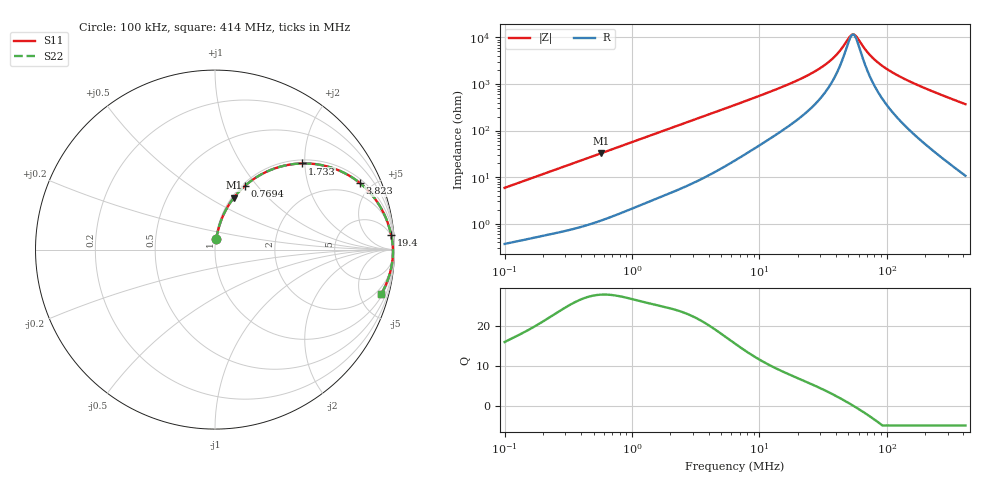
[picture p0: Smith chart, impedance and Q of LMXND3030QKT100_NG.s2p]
! LMXND3030QKT100_NG  S-PARAMETER MODEL  ( General Type )
! Model Generated by TAIYO YUDEN Corporation (https://www.yuden.co.jp/en/)
! Version 1.0
! TAIYO YUDEN Control No. 191023NI43SB-FBB
! Copyright(c) 2019 TAIYO YUDEN CO.,LTD. All Rights Reserved.
! Product Description (link to TY-COMPAS)
! https://ds.yuden.co.jp/TYCOMPAS/or/detail?pn=LMXND3030QKT100MNG&u=M
! Products Name : Inductors
! Characteristics :
!  Inductance : 10 uH , SRF(min) : 28 MHz , DC Resistance(max) : 0.264 Ohm
!  Rated Current : Saturation :700 mA , Temp Rise : 710 mA (40 degC)
!  Case Size : 3.0 x 3.0 / 0.118 x 0.118 [mm/inch] , Thickness : 1.5 / 0.059 [mm/inch]
!  (Conditions: Temperature = 25 degC , DC Bias Current/Voltage = 0A / 0V)
! External Node Assignments :
!  1  o---GGG---o  2
! GND o---------o GND
! Frequency Range : 0.1MHz  -  413.982163MHz  [ 402 STEP ]
# MHz S RI R 50
! Freq[MHz].  S11 Real  S11 Imag  S21 Real  S21 Imag  S12 Real  S12 Imag  S22 Real  S22 Imag
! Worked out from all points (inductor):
!   401 points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, 100 kHz to 414 MHz, reference 50 ohm
!   read as one part in series: L = 9.29 uH near 104.3 kHz
!   highest Q = 27.9 at 574.9 kHz (marker M1), where L = 9.05 uH
!   self-resonance near 53.8 MHz
!   S11 on the Smith chart (normalised r, x): 100 kHz: 1.01, +0.12; 769.4 kHz: 1.03, +0.87; 1.733 MHz: 1.08, +1.93; 3.823 MHz: 1.20, +4.22; 19.4 MHz: 4, +23; 414 MHz: 1.21, -7.38
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0.1  0.00706 0.0581  0.9929 -0.0581  0.9929 -0.0581  0.00706 0.0581
0.211606  0.0201 0.1191  0.9799 -0.1191  0.9799 -0.1191  0.0201 0.1191
0.403501  0.0578 0.2154  0.9422 -0.2154  0.9422 -0.2154  0.0578 0.2154
0.574865  0.105 0.2891  0.895 -0.2891  0.895 -0.2891  0.105 0.2891
0.769415  0.1684 0.3565  0.8316 -0.3565  0.8316 -0.3565  0.1684 0.3565
1.628129  0.4542 0.4784  0.5458 -0.4784  0.5458 -0.4784  0.4542 0.4784
1.73307  0.4835 0.4801  0.5165 -0.4801  0.5165 -0.4801  0.4835 0.4801
2.469096  0.6461 0.4574  0.3539 -0.4574  0.3539 -0.4574  0.6461 0.4574
3.823222  0.8053 0.3724  0.1947 -0.3724  0.1947 -0.3724  0.8053 0.3724
6.434145  0.9128 0.2518  0.0872 -0.2518  0.0872 -0.2518  0.9128 0.2518
19.39728  0.9811 0.0826  0.0189 -0.0826  0.0189 -0.0826  0.9811 0.0826
25.96183  0.9863 0.0555  0.0137 -0.0555  0.0137 -0.0555  0.9863 0.0555
37.76586  0.99 0.0259  0.00999 -0.0259  0.00999 -0.0259  0.99 0.0259
42.79117  0.9907 0.0168  0.00928 -0.0168  0.00928 -0.0168  0.9907 0.0168
50.54681  0.9913 0.00502  0.00868 -0.00502  0.00868 -0.00502  0.9913 0.00502
53.80481  0.9915 0.000618  0.00855 -0.000618  0.00855 -0.000618  0.9915 0.000618
58.47779  0.9916 -0.00527  0.00845 0.00527  0.00845 0.00527  0.9916 -0.00527
69.07654  0.9915 -0.0172  0.00851 0.0172  0.00851 0.0172  0.9915 -0.0172
78.26819  0.9912 -0.0265  0.0088 0.0265  0.0088 0.0265  0.9912 -0.0265
104.7562  0.9896 -0.05  0.0104 0.05  0.0104 0.05  0.9896 -0.05
183.7917  0.9802 -0.1086  0.0198 0.1086  0.0198 0.1086  0.9802 -0.1086
413.9822  0.9253 -0.2487  0.0747 0.2487  0.0747 0.2487  0.9253 -0.2487
